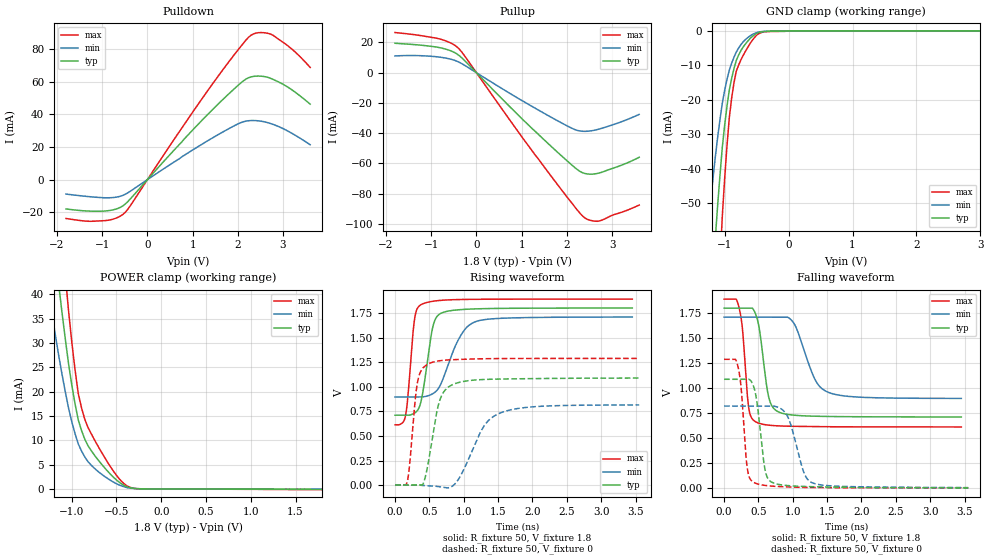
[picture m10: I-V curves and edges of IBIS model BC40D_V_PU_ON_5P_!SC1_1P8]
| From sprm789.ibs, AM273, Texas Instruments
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|   Model Cell BC40D_V_PU_ON_5P_!SC1_1P8
|BC40D_V_PU_ON_5P_!SC1_1P8
[Model]   BC40D_V_PU_ON_5P_!SC1_1P8
Model_type   I/O
Polarity   Non-Inverting
Enable   Active-Low
Vinl =  0.63
Vinh =  1.17
Cref =  15pF
Rref =  100.0000M
Vref =  0V
Vmeas =  0.9
C_comp   2.233931p   2.204415p   2.290246p
|[Input load] weak_pu_on
|[Output drive] fast
|[supplytol] 5
|[temp] ind
[Model Spec]
Vinl   0.63   0.5985   0.6615
Vinh   1.17   1.1115   1.2285
[Temperature Range]   25   125   -40
[Voltage Range]   1.8   1.71   1.89
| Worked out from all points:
|   slope of the pulldown table from 0 to 0.27 V, typ, clamps not added: 32.2 ohm
|   slope of the pullup table from 0 to 0.27 V, typ, clamps not added: 32.5 ohm
|   GND clamp passes 1 mA (typ) near -0.52 V on its own axis
|   POWER clamp passes 1 mA (typ) near -0.44 V on its own axis
|   rising waveform, R_fixture 50, V_fixture 1.8: 20-80 % time 141ps typ, 293ps min, 91.4ps max; typ from 0.711 V to 1.8 V
|   rising waveform, R_fixture 50, V_fixture 0: 20-80 % time 174ps typ, 351ps min, 104ps max; typ from 0.002 V to 1.09 V
|   falling waveform, R_fixture 50, V_fixture 1.8: 20-80 % time 128ps typ, 263ps min, 86.1ps max; typ from 1.8 V to 0.711 V
|   falling waveform, R_fixture 50, V_fixture 0: 20-80 % time 111ps typ, 195ps min, 82.6ps max; typ from 1.09 V to 0.002 V
| Nom Voltages:
|   VDD=1.1, VDDS=1.8, VDDS18=1.8, ESD_BIASFET=0, VSS=0, VSSS=0
| Min Voltages:
|   VDD=1.045, VDDS=1.71, VDDS18=1.71, ESD_BIASFET=0, VSS=0, VSSS=0
| Max Voltages:
|   VDD=1.16, VDDS=1.89, VDDS18=1.89, ESD_BIASFET=0, VSS=0, VSSS=0
[POWER_clamp]
|   voltage   I(typ)   I(min)   I(max)
-1.8V     158.8mA    112.5mA    219.8mA
-1.255V   59.97mA    40.01mA    84.91mA
-1.145V   41.92mA    27.41mA    59.76mA
-1.109V   36.32mA    23.62mA    51.83mA
-1.073V   30.96mA    20.04mA    44.16mA
-1.036V   25.83mA    16.67mA    36.76mA
-963.6mV  17.54mA    11.39mA    24.56mA
-890.9mV  12.01mA    7.798mA    16.67mA
-818.2mV  8.875mA    5.598mA    12.64mA
-563.6mV  2.954mA    1.726mA    4.46mA
-272.7mV  55.97uA    39.54uA    57.56uA
1.8V      -99.94uA   -59.14uA   -145.1uA
[Pulldown]
|   voltage   I(typ)   I(min)   I(max)
-1.8V     -17.92mA   -8.85mA    -23.8mA
-1.309V   -19.26mA   -10.37mA   -25.51mA
-927.3mV  -19.22mA   -11.12mA   -25.08mA
-654.5mV  -17.65mA   -10.56mA   -23.13mA
-490.9mV  -14.97mA   -8.985mA   -20.05mA
1.364V    40.78mA    24.32mA    55.7mA
2.073V    59.41mA    35mA       81.9mA
2.291V    62.96mA    36.2mA     88.48mA
2.509V    63.41mA    35.84mA    90.12mA
2.782V    61.38mA    33.82mA    88.42mA
3.218V    54.59mA    28.02mA    79.45mA
3.6V      46.26mA    21.39mA    68.79mA
[Pullup]
|   voltage   I(typ)   I(min)   I(max)
-1.8V     19.47mA    11.11mA    26.55mA
-818.2mV  16.61mA    10.32mA    22.37mA
-545.5mV  14.21mA    8.765mA    19.31mA
-381.8mV  11.35mA    6.928mA    15.71mA
1.255V    -37.58mA   -22.7mA    -52.59mA
2.127V    -61.49mA   -36.97mA   -86.91mA
2.291V    -65.3mA    -38.55mA   -92.97mA
2.4V      -66.65mA   -38.77mA   -96.07mA
2.564V    -67.08mA   -38.3mA    -97.93mA
2.727V    -66.24mA   -37.15mA   -97.99mA
3.273V    -60.4mA    -31.68mA   -91.65mA
3.6V      -55.92mA   -27.55mA   -87.52mA
[GND_clamp]
|   voltage   I(typ)   I(min)   I(max)
-1.8V     -270.2mA   -170.2mA   -430.1mA
-1.255V   -91.68mA   -55.92mA   -148.5mA
-1.145V   -59.94mA   -36.46mA   -97.14mA
-1.109V   -50.51mA   -30.84mA   -81.61mA
-1.073V   -41.77mA   -25.67mA   -67.13mA
-1.036V   -33.71mA   -20.95mA   -53.68mA
-927.3mV  -17.15mA   -11.38mA   -25.19mA
-854.5mV  -10.96mA   -7.663mA   -15.08mA
-781.8mV  -7.031mA   -5.001mA   -9.947mA
-563.6mV  -1.569mA   -1.041mA   -2.641mA
-18.18mV  0A         0A         0A
3.6V      0A         0A         0A
[Ramp]
| variable   typ   min   max
dV/dt_f 0.66507934/0.13047563n 0.49947306/0.26909371n 0.77654614/87.861951p
dV/dt_r 0.66370141/0.17654672n 0.50912868/0.36419589n 0.78039356/0.10498627n
R_load = 50
[Rising Waveform]
R_fixture = 50
V_fixture = 1.8
V_fixture_min = 1.71
V_fixture_max = 1.89
|   time   V(typ)   V(min)   V(max)
0s        710.6mV    895.2mV    613mV
149.8ps   710.6mV    895.2mV    696.6mV
183.7ps   710.6mV    895.2mV    877.5mV
284.2ps   732.1mV    895.2mV    1.689V
384.1ps   869.5mV    896.4mV    1.836V
548.5ps   1.604V     928.8mV    1.868V
678.4ps   1.749V     1.045V     1.878V
943.6ps   1.783V     1.505V     1.886V
1.179ns   1.791V     1.663V     1.888V
3.453ns   1.8V       1.708V     1.89V
[Rising Waveform]
R_fixture = 50
V_fixture = 0
V_fixture_min = 0
V_fixture_max = 0
|   time   V(typ)   V(min)   V(max)
0s        2.151mV    0V         3.038mV
177.5ps   2.151mV    0V         34.93mV
323.4ps   2.151mV    0V         1.032V
404.2ps   7.379mV    -3.367mV   1.188V
483.3ps   228mV      -6.923mV   1.232V
647.8ps   855.9mV    -16.03mV   1.264V
857.4ps   1.027V     2.586mV    1.275V
1.281ns   1.073V     585.4mV    1.284V
1.514ns   1.078V     728.1mV    1.286V
3.554ns   1.088V     815mV      1.288V
[Falling Waveform]
R_fixture = 50
V_fixture = 1.8
V_fixture_min = 1.71
V_fixture_max = 1.89
|   time   V(typ)   V(min)   V(max)
0s        1.8V       1.71V      1.89V
215ps     1.8V       1.71V      1.814V
269.6ps   1.8V       1.71V      1.578V
357.6ps   1.8V       1.71V      808.4mV
468ps     1.724V     1.71V      660.2mV
646.5ps   919.7mV    1.71V      629.7mV
789.1ps   763.1mV    1.71V      622.3mV
1.018ns   729.3mV    1.647V     617.9mV
1.502ns   716.5mV    962.7mV    613.8mV
3.453ns   711.4mV    897.1mV    611.7mV
[Falling Waveform]
R_fixture = 50
V_fixture = 0
V_fixture_min = 0
V_fixture_max = 0
|   time   V(typ)   V(min)   V(max)
0s        1.089V     820.4mV    1.288V
199.2ps   1.089V     820.4mV    1.225V
249.5ps   1.089V     820.4mV    995mV
337.2ps   1.089V     820.4mV    202.8mV
438.5ps   998.1mV    820.4mV    54.99mV
592.1ps   199.6mV    820.4mV    26.96mV
703.1ps   56.11mV    820.4mV    19.3mV
920ps     25.47mV    722.5mV    12.07mV
1.285ns   13.94mV    52.56mV    5.243mV
3.554ns   2.463mV    4.989mV    2.437mV
